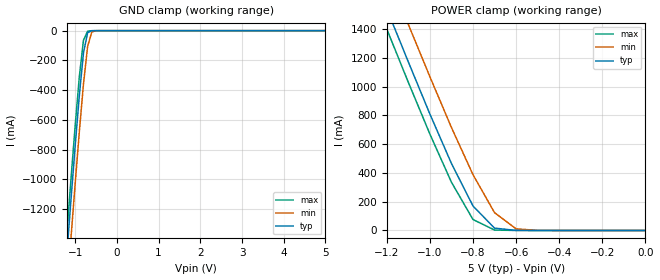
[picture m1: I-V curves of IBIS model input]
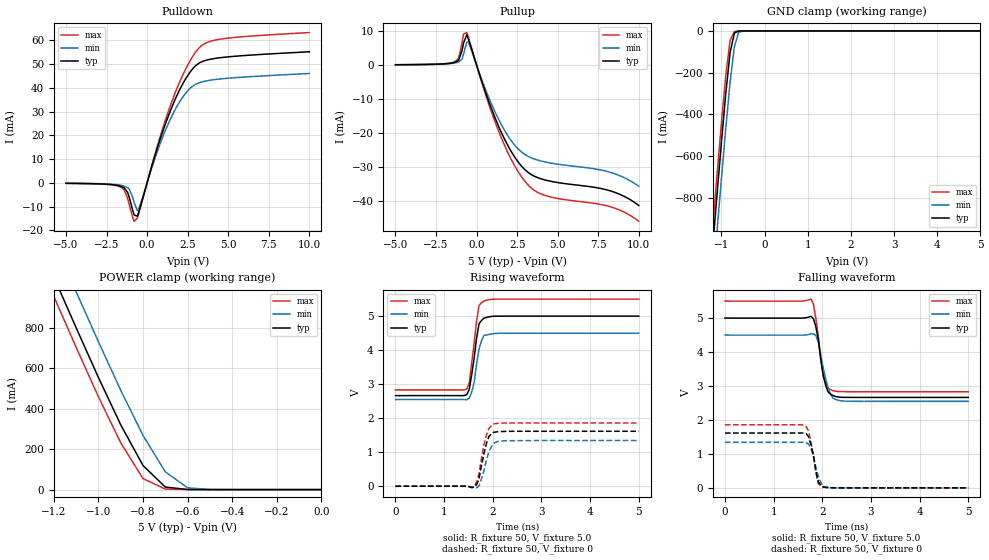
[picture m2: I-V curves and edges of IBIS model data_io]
| SOJ  Package & Commercial  operation.
[IBIS Ver]   3.2
[Comment Char]   |_char
[File name]   as7c256a_sojc.ibs
[File Rev]   1.0
[Date]   Apr 8, 2005 2:44:33 PM
[Source]
Alliance Semiconductor Corporation
[Notes]
This model  is for SOJ package & Commercial operation.
[Disclaimer]
Data is for modeling purpose only and is not guaranted.
This IBIS model is provided on an "AS IS" basis and Alliance Semiconductor makes
absolutely no warranty with respect to the information contained
herein.The entire risk as to quality and performance
is with the Customer. ACCORDINGLY, IN NO EVENT SHALL THE COMPANY BE
LIABLE FOR ANY DAMAGES, WHETHER IN CONTRACT OR TORT,INCLUDING ANY
LOST PROFITS OR OTHER INCIDENTAL, CONSEQUENTIAL, EXEMPLARY, OR
PUNITIVE DAMAGES ARISING OUT OF THE USE OR APPLICATION OF THE IBIS
model provided in this package.
[Copyright]
Alliance Semiconductor Corporation
| SOJ Package & Commercial  operation.
[Component]   AS7C256A_SOJC
Si_location Pin
Timing_location Pin
[Manufacturer]   Alliance Semiconductor Corporation
[Package]
R_pkg   158.885m   88.47m   229.3m
L_pkg   7.1455nH   4.457nH   9.834nH
C_pkg   1.118pF   0.777pF   1.459pF
[Pin] signal_name   model_name
1   A14   input
2   A12   input
3   A7   input
4   A6   input
5   A5   input
6   A4   input
7   A3   input
8   A2   input
9   A1   input
10   A0   input
11   IO0   data_io
12   IO1   data_io
13   IO2   data_io
14   GND   GND
15   IO3   data_io
16   IO4   data_io
17   IO5   data_io
18   IO6   data_io
19   IO7   data_io
20   NCE   input
21   A10   input
22   NOE   input
23   A11   input
24   A9   input
25   A8   input
26   A13   input
27   NWE   input
28   VCC   POWER
| Models and submodels in the file (2): input (Input), data_io (I/O)
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[Model]   input
Model_type Input
Vinh=2.2V
Vinl=0.8V
C_comp   4pF   4pF   4pF
[Model Spec]
[Temperature Range] 25   70   0
[Voltage Range]   5.0   4.5   5.5
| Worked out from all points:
|   GND clamp passes 1 mA (typ) near -0.60 V on its own axis
|   POWER clamp passes 1 mA (typ) near -0.60 V on its own axis
[GND Clamp]
-5V       -15.51A    -15.6A     -15.47A
-1.2V     -1.509A    -1.76A     -1.371A
-1.1V     -1.14A     -1.396A    -1.001A
-1V       -779.5mA   -1.033A    -643.1mA
-900mV    -438.9mA   -682.6mA   -312mA
-800mV    -150.4mA   -359mA     -64.57mA
-700mV    -13.19mA   -105.3mA   -3.183mA
-600mV    -657.5uA   -8.634mA   -287.1uA
-500mV    -49.35uA   -401uA     -23.43uA
5V        149.8pA    470.6uA    109.2pA
[POWER Clamp]
-5V       15.54A     15.63A     15.49A
-1.2V     1.539A     1.796A     1.399A
-1.1V     1.171A     1.432A     1.029A
-1V       809mA      1.068A     669.6mA
-900mV    465.4mA    715.5mA    335.2mA
-800mV    170mA      387.4mA    76.06mA
-700mV    16.13mA    123.8mA    3.007mA
-600mV    564.2uA    11.16mA    165.7uA
-500mV    33.62uA    470.6uA    13.97uA
0V        149.8pA    622pA      136.6pA
[Model]   data_io
Model_type I/O
Enable Active-High
Polarity Non-Inverting
Vinh=2.2V
Vinl=0.8V
Vref=1.72V
Vmeas=1.5V
Rref=168
Cref=30pF
C_comp   4pF   4pF   4pF
[Temperature Range] 25   70   0
[Voltage Range]   5.0   4.5   5.5
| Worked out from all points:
|   slope of the pulldown table from 0 to 0.75 V, typ, clamps not added: 43.6 ohm
|   slope of the pullup table from 0 to 0.75 V, typ, clamps not added: 70.1 ohm
|   GND clamp passes 1 mA (typ) near -0.60 V on its own axis
|   POWER clamp passes 1 mA (typ) near -0.60 V on its own axis
|   falling waveform, R_fixture 50, V_fixture 5.0: 20-80 % time 154ps typ, 178ps min, 145ps max; typ from 5 V to 2.66 V
|   falling waveform, R_fixture 50, V_fixture 0: 20-80 % time 133ps typ, 154ps min, 135ps max; typ from 1.61 V to 0.003 V
|   rising waveform, R_fixture 50, V_fixture 5.0: 20-80 % time 139ps typ, 136ps min, 135ps max; typ from 2.66 V to 5 V
|   rising waveform, R_fixture 50, V_fixture 0: 20-80 % time 148ps typ, 163ps min, 150ps max; typ from 0 V to 1.62 V
[Pullup]
-5V       100uA      90uA       100uA
-1.4V     732uA      552uA      875uA
-1.1V     1.496mA    945uA      2.136mA
-900mV    4.264mA    1.739mA    6.423mA
-800mV    6.548mA    3.333mA    9.146mA
-600mV    8.924mA    6.727mA    9.574mA
1.4V      -18.49mA   -16.39mA   -19.94mA
2.3V      -26.74mA   -23.29mA   -29.25mA
3.2V      -31.71mA   -26.94mA   -35.45mA
4.5V      -34.16mA   -28.81mA   -38.77mA
8V        -36.73mA   -31.28mA   -41.42mA
10V       -41.35mA   -35.69mA   -46.02mA
[Pulldown]
-5V       -210uA     -190uA     -220uA
-1.5V     -1.796mA   -1.198mA   -2.364mA
-1.2V     -4.044mA   -2.081mA   -6.59mA
-800mV    -13.5mA    -8.279mA   -16.2mA
-600mV    -14.07mA   -11.7mA    -14.85mA
-500mV    -11.96mA   -10.83mA   -12.53mA
800mV     18.25mA    16.38mA    19.34mA
1.7V      34.67mA    30.45mA    37.33mA
2.6V      46.15mA    39.44mA    50.77mA
3.2V      50.36mA    42.08mA    56.77mA
4.7V      52.81mA    43.85mA    60.66mA
10V       55.16mA    46mA       63.25mA
[GND Clamp]
-5V       -10.56A    -10.63A    -10.53A
-1.2V     -1.03A     -1.202A    -935.9mA
-1.1V     -779.5mA   -954.3mA   -684.6mA
-1V       -534.1mA   -707.4mA   -441mA
-900mV    -302.3mA   -468.7mA   -215.6mA
-800mV    -105.5mA   -248.2mA   -46.47mA
-700mV    -10.47mA   -74.84mA   -2.861mA
-600mV    -637.4uA   -7.115mA   -283.5uA
-500mV    -49.22uA   -392.2uA   -23.4uA
5V        149.8pA    458.3uA    109.2pA
[POWER Clamp]
-5V       10.58A     10.65A     10.55A
-1.2V     1.051A     1.226A     955.3mA
-1.1V     800.4mA    978.3mA    703.7mA
-1V       554.1mA    731.1mA    459mA
-900mV    320.3mA    491mA      231.4mA
-800mV    118.9mA    267.6mA    54.28mA
-700mV    12.55mA    87.52mA    2.669mA
-600mV    546.8uA    8.999mA    164.6uA
-500mV    33.56uA    458.2uA    13.96uA
0V        149.8pA    622pA      136.6pA
[Falling Waveform]
R_fixture=50
V_fixture=5.0
V_fixture_min=4.5
V_fixture_max=5.5
0s        5V         4.5V       5.5V
1.768ns   5.05V      4.534V     5.555V
1.818ns   4.979V     4.529V     5.413V
1.869ns   4.736V     4.479V     4.976V
1.919ns   4.362V     4.297V     4.454V
1.97ns    3.773V     3.899V     3.793V
2.02ns    3.304V     3.529V     3.308V
2.121ns   2.822V     2.937V     2.939V
2.222ns   2.716V     2.639V     2.862V
5ns       2.663V     2.548V     2.831V
[Falling Waveform]
R_fixture=50
V_fixture=0
V_fixture_min=0
V_fixture_max=0
0s        1.615V     1.342V     1.858V
1.566ns   1.618V     1.344V     1.862V
1.667ns   1.603V     1.338V     1.811V
1.717ns   1.512V     1.287V     1.674V
1.768ns   1.27V      1.148V     1.35V
1.818ns   950.5mV    941.5mV    961.9mV
1.869ns   495.1mV    614.9mV    458mV
1.919ns   177.8mV    343.7mV    122.5mV
2.02ns    26.62mV    46.75mV    21.71mV
5ns       2.644mV    2.564mV    2.869mV
[Rising Waveform]
R_fixture=50
V_fixture=5.0
V_fixture_min=4.5
V_fixture_max=5.5
0s        2.663V     2.547V     2.83V
1.465ns   2.693V     2.543V     2.853V
1.515ns   2.84V      2.591V     3.037V
1.566ns   3.272V     2.76V      3.607V
1.616ns   3.756V     3.049V     4.202V
1.667ns   4.349V     3.593V     4.854V
1.717ns   4.773V     4.033V     5.31V
1.818ns   4.938V     4.43V      5.442V
2.222ns   4.997V     4.496V     5.496V
5ns       4.997V     4.497V     5.496V
[Rising Waveform]
R_fixture=50
V_fixture=0
V_fixture_min=0
V_fixture_max=0
0s        0V         0V         0V
1.616ns   -27.22mV   -32.91mV   -16.82mV
1.667ns   45.73mV    -45.67mV   122.8mV
1.717ns   225.1mV    15.94mV    371.5mV
1.818ns   962.6mV    463.4mV    1.225V
1.869ns   1.252V     768mV      1.498V
1.919ns   1.461V     1.013V     1.698V
2.02ns    1.587V     1.262V     1.833V
2.273ns   1.612V     1.338V     1.859V
5ns       1.616V     1.343V     1.859V
[Ramp]
R_load=50
dV/dt_r   9.695E-1/1.457E-10   8.059E-1/1.613E-10   1.116E+0/1.495E-10
dV/dt_f   1.402E+0/1.459E-10   1.171E+0/1.780E-10   1.602E+0/1.376E-10
|[End   data_io
